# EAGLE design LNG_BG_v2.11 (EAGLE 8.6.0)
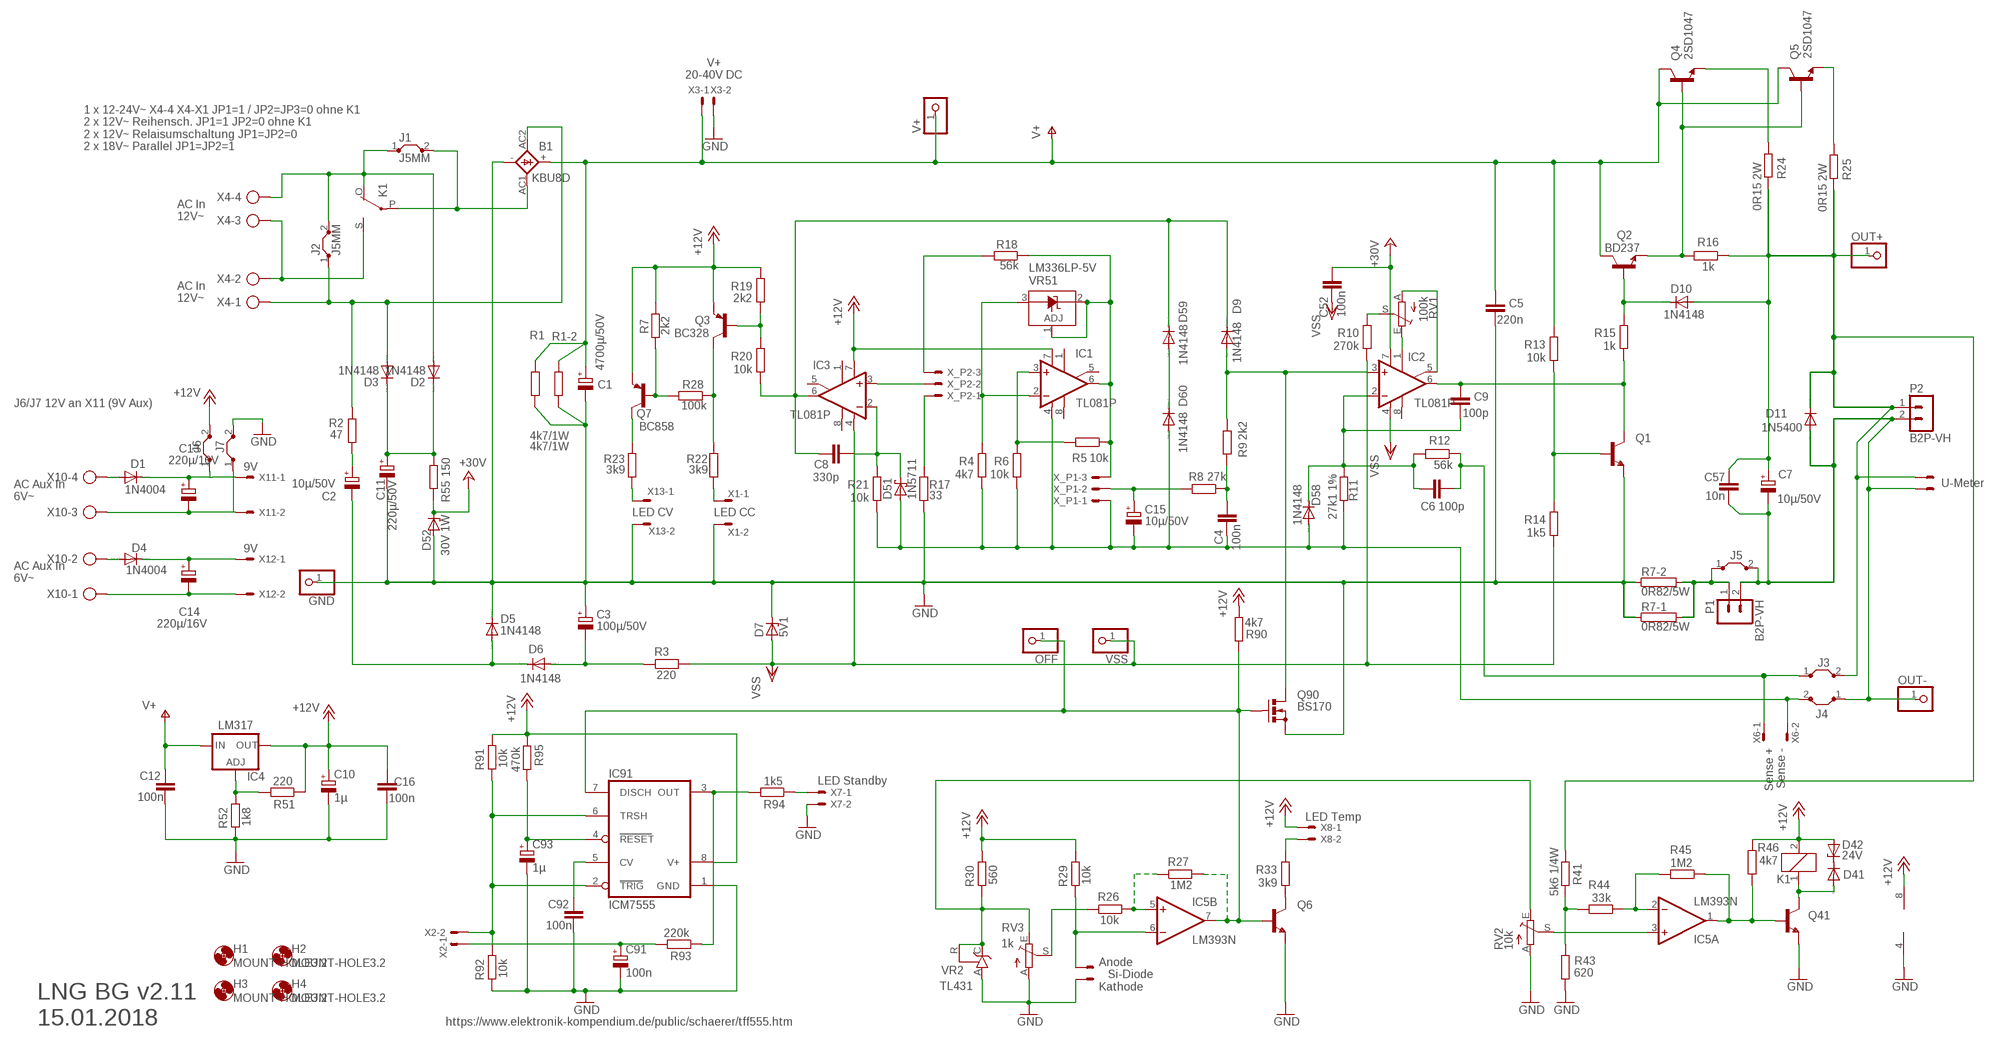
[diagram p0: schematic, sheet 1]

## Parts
B1  KBU8D  GBU4  [GBU4S]
C1  4700µ/50V  CPOL-EUE10-25  [EB25D]
C2  10µ/50V  CPOL-EUE2.5-6  [E2,5-6]
C3  100µ/50V  CPOL-EUE2.5-6  [E2,5-6]
C4  100n  C-EU050-024X044  [C050-024X044]
C5  220n  C-EUC1206  [C1206]
C6  100p  C-EU050-024X044  [C050-024X044]
C7  10µ/50V  CPOL-EUE2.5-6  [E2,5-6]
C8  330p  C-EU050-024X044  [C050-024X044]
C9  100p  C-EU050-024X044  [C050-024X044]
C10  1µ  CPOL-EUE1.8-4  [E1,8-4]
C11  220µ/50V  CPOL-EUE5-10.5  [E5-10,5]
C12  100n  C-EUC0805K  [C0805K]
C13  220µ/16V  CPOL-EUE3.5-8  [E3,5-8]
C14  220µ/16V  CPOL-EUE3.5-8  [E3,5-8]
C15  10µ/50V  CPOL-EUE2.5-6  [E2,5-6]
C16  100n  C-EUC0805  [C0805]
C52  100n  C-EUC0805  [C0805]
C57  10n  C-EUC1206  [C1206]
C91  100n  CPOL-EUE1.8-4  [E1,8-4]
C92  100n  C-EUC0805  [C0805]
C93  1µ  CPOL-EUE1.8-4  [E1,8-4]
D1  1N4004  [DO41-10]
D2  1N4148  1N4004  [DO41-10]
D3  1N4148  1N4004  [DO41-10]
D4  1N4004  [DO41-10]
D5  1N4148  1N4148DO35-10  [DO35-10]
D6  1N4148  1N4148DO35-10  [DO35-10]
D7  5V1  BZV10  [DO34Z7]
D9  1N4148  1N4148DO35-10  [DO35-10]
D10  1N4148  1N4148DO35-10  [DO35-10]
D11  1N5400  [DO201-15]
D41  ES2D  [SMB]
D42  24V  ZENER-DIODESOD80C  [SOD80C]
D51  1N5711  SCHOTTKY-DIODEDO35-7  [DO35-7]
D52  30V 1W  ZPY  [DO41Z10]
D58  1N4148  1N4148DO35-10  [DO35-10]
D59  1N4148  1N4148DO35-10  [DO35-10]
D60  1N4148  1N4148DO35-10  [DO35-10]
GND  PINHD-1X1  [1X01]
H1  MOUNT-HOLE3.2  [3,2]
H2  MOUNT-HOLE3.2  [3,2]
H3  MOUNT-HOLE3.2  [3,2]
H4  MOUNT-HOLE3.2  [3,2]
IC1  TL081P  [DIL08]
IC2  TL081P  [DIL08]
IC3  TL081P  [DIL08]
IC4  LM317  LM317TS  [317TS]
IC5  LM393N  [DIL08]
IC91  ICM7555  [DIL08]
J1  J5MM  [05]
J2  J5MM  [05]
J3  J5MM  [05]
J4  J5MM  [05]
J5  J5MM  [05]
J6  J5MM  [05]
J7  J5MM  [05]
K1  G6RW  [G6RW]
OFF  PINHD-1X1  [1X01]
OUT+  PINHD-1X1  [1X01]
OUT-  PINHD-1X1  [1X01]
P1  B2P-VH  [B2P-VH]
P2  B2P-VH  [B2P-VH]
Q1  BC337-NPN-TO92-CBE  [TO92-CBE]
Q2  BD237  -NPN-TO126V  [TO126V]
Q3  BC328  [TO92-EBC]
Q4  2SD1047  2SC3855  [SC-65]
Q5  2SD1047  2SC3855  [SC-65]
Q6  BC337-NPN-TO92-CBE  [TO92-CBE]
Q7  BC858  BC858ALT1SMD  [SOT23-BEC]
Q41  BC337-NPN-TO92-CBE  [TO92-CBE]
Q90  BS170  [SOT54E]
R1  4k7/1W  R-EU_R2512  [R2512]
R1-2  4k7/1W  R-EU_R2512  [R2512]
R2  47  R-EU_0411/15  [0411/15]
R3  220  R-EU_0207/10  [0207/10]
R4  4k7  R-EU_0207/10  [0207/10]
R5  10k  R-EU_0207/10  [0207/10]
R6  10k  R-EU_0207/10  [0207/10]
R7  2k2  R-EU_R1206  [R1206]
R7-1  0R82/5W  RKH208-8  [KH208-8]
R7-2  0R82/5W  RKH208-8  [KH208-8]
R8  27k  R-EU_0207/10  [0207/10]
R9  2k2  R-EU_0207/10  [0207/10]
R10  270k  R-EU_0207/10  [0207/10]
R11  27k1 1%  R-EU_0207/10  [0207/10]
R12  56k  R-EU_0207/10  [0207/10]
R13  10k  R-EU_0207/10  [0207/10]
R14  1k5  R-EU_0207/10  [0207/10]
R15  1k  R-EU_0207/10  [0207/10]
R16  1k  R-EU_0207/10  [0207/10]
R17  33  R-EU_0207/10  [0207/10]
R18  56k  R-EU_0207/10  [0207/10]
R19  2k2  R-EU_0207/10  [0207/10]
R20  10k  R-EU_0207/10  [0207/10]
R21  10k  R-EU_0207/10  [0207/10]
R22  3k9  R-EU_0207/10  [0207/10]
R23  3k9  R-EU_0207/10  [0207/10]
R24  0R15 2W  R-EU_0617/5V  [0617V]
R25  0R15 2W  R-EU_0617/5V  [0617V]
R26  10k  R-EU_0207/10  [0207/10]
R27  1M2  R-EU_0207/10  [0207/10]
R28  100k  R-EU_R1206  [R1206]
R29  10k  R-EU_0207/10  [0207/10]
R30  560  R-EU_0207/10  [0207/10]
R33  3k9  R-EU_0207/10  [0207/10]
R41  5k6 1/4W  R-EU_0207/10  [0207/10]
R43  620  R-EU_0207/10  [0207/10]
R44  33k  R-EU_0207/10  [0207/10]
R45  1M2  R-EU_0207/10  [0207/10]
R46  4k7  R-EU_0207/10  [0207/10]
R51  220  R-EU_0207/10  [0207/10]
R52  1k8  R-EU_0207/10  [0207/10]
R55  150  R-EU_0207/10  [0207/10]
R90  4k7  R-EU_0207/10  [0207/10]
R91  10k  R-EU_0207/10  [0207/10]
R92  10k  R-EU_0207/10  [0207/10]
R93  220k  R-EU_0207/10  [0207/10]
R94  1k5  R-EU_0207/10  [0207/10]
R95  470k  R-EU_0207/10  [0207/10]
RV1  100k  TRIM_EU-B64Y  [B64Y]
RV2  10k  TRIM_EU-B64Y  [B64Y]
RV3  1k  TRIM_EU-B64Y  [B64Y]
U_METER  U-Meter  22-23-2021  [22-23-2021]
V+  PINHD-1X1  [1X01]
VR2  TL431  TL431CLP  [TO92-CLP]
VR51  LM336LP-5V  LM336LP  [TO92]
VSS  PINHD-1X1  [1X01]
X1  LED CC  22-23-2021  [22-23-2021]
X2  PSK-2  22-23-2021  [22-23-2021]
X3  PSK-2  22-23-2021  [22-23-2021]
X4  AK500/4  [AK500/4]
X5  PSK-2  22-23-2021  [22-23-2021]
X6  22-23-2021  [22-23-2021]
X7  LED Standby  22-23-2021  [22-23-2021]
X8  LED Temp  22-23-2021  [22-23-2021]
X10  AK500/4  [AK500/4]
X11  9V  22-23-2021  [22-23-2021]
X12  9V  22-23-2021  [22-23-2021]
X13  LED CV  22-23-2021  [22-23-2021]
X_P1  22-23-2031  [22-23-2031]
X_P2  22-23-2031  [22-23-2031]

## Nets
+12V: C10.+ C16.1 D42.A IC1.7(V+) IC3.7(V+) IC4.2(OUT) IC5.8(P:V+) IC91.8(V+) J6.2 K1.2 Q3.E Q7.E R7.1 R19.2 R29.2 R30.2 R46.2 R51.1 R90.1 R91.2 R95.1 X8.1
+24V: C52.1 D52.C IC2.7(V+) R55.1 ; supply symbol labelled +30V
AC2-1: K1.S(2:S) X4.2 X4.3
AC2-2: B1.AC2(AC1) D3.A J2.1 R2.1 X4.1
GND: B1.- C1.- C3.+ C5.2 C10.- C11.- C12.2 C16.2 C91.- C92.2 C93.- D5.C D7.C D52.A GND.1 IC5.4(P:V-) IC91.1(GND) J7.2 Q1.E Q6.E Q41.E Q90.S R1-2.1 R1.1 R7-1.1 R7-2.1 R17.1 R43.1 R52.1 R92.1 RV2.A RV3.A VR2.A X1.2 X3.2 X5.2 X7.2 X13.2
N$1: IC91.3(OUT) R93.1 R94.2
N$2: R94.1 X7.1
N$3: C2.+ R2.2
N$4: B1.AC1(AC2) J1.2 K1.P(2:P)
N$5: C2.- D5.A D6.C
N$6: Q3.B R19.1 R20.2
N$7: C3.- D6.A R3.1
N$8: D59.A D60.C
N$9: C8.2 D9.C D59.C IC3.6(OUT) R20.1
N$10: C8.1 D51.C IC3.2(-IN) R21.2
N$11: R22.1 X1.1
N$12: Q3.C R22.2 R28.1
N$13: C11.+ D2.C D3.C R55.2
N$14: IC3.3(+IN) X_P2.2
N$15: R17.2 X_P2.1
N$16: R18.2 X_P2.3
N$17: IC1.3(+IN) R5.2 R6.2
N$18: R41.1 R43.2 R44.2
N$19: IC1.2(-IN) R4.2 VR51.3(A)
N$20: J5.1 P1.1 R7-1.2 R7-2.2
N$21: C4.1 R8.1 R9.2
N$22: D9.A IC2.3(+IN) Q90.D R9.1
N$23: C93.+ IC91.4(RESET) R95.2
N$24: R10.2 RV1.S
N$25: IC2.1(ON1) RV1.E
N$26: IC2.5(ON2) RV1.A
N$27: C9.1 IC2.6(OUT) Q1.C R15.1
N$28: Q1.B R13.1 R14.2
N$29: D10.C Q2.3(B) R15.2
N$30: IC5.2(A:-IN) R44.1 R45.2
N$31: IC5.5(B:+IN) R26.2 R27.1
N$32: IC91.2(TRIG) IC91.6(TRSH) R91.1 R92.2 X2.2
N$33: IC5.3(A:+IN) RV2.S
N$34: C15.+ R8.2 X_P1.2
N$35: C6.1 C9.2 D58.C IC2.2(-IN) R11.2 R12.2
N$36: C92.1 IC91.5(CV)
N$37: IC5.6(B:-IN) R29.1 X5.1
N$38: R33.2 X8.2
N$39: IC5.1(A:OUT) Q41.B R45.1 R46.1
N$40: R30.1 RV2.E RV3.E VR2.C VR2.R
N$41: D41.A K1.1 Q41.C
N$42: Q4.3(E) R24.2
N$43: C13.+ D1.C J6.1 X11.1
N$44: IC4.1(ADJ) R51.2 R52.2
N$45: R26.1 RV3.S
N$46: D2.A J1.1 J2.2 K1.O(2:O) X4.4
N$47: Q5.3(E) R25.2
N$48: R23.1 X13.1
N$49: Q7.B R7.2 R28.2
N$50: Q2.1(E) Q4.1(B) Q5.1(B) R16.2
N$51: C14.+ D4.C X12.1
N$52: D1.A X10.4
N$53: C91.+ R93.2 X2.1
N$54: Q7.C R23.2
N$55: D4.A X10.2
N$56: Q6.C R33.1
N$57: C13.- J7.1 X10.3 X11.2
N$59: C14.- X10.1 X12.2
N$60: D41.C D42.C
OUT+: C7.+ C57.2 D10.A D11.C J3.2 OUT+.1 P2.1 R16.1 R24.1 R25.1 R41.2 U_METER.1
OUT-: C7.- C57.1 D11.A J4.1 J5.2 OUT-.1 P1.2 P2.2 U_METER.2
SENSE+: C6.2 J3.1 R12.1 X6.1
SENSE-: C4.2 C15.- D51.A D58.A D60.A IC1.4(V-) J4.2 R4.1 R6.1 R11.1 R21.1 X6.2 X_P1.1
SHUTDOWN: IC5.7(B:OUT) IC91.7(DISCH) OFF.1 Q6.B Q90.G R27.2 R90.2
V+: B1.+ C1.+ C5.1 C12.1 IC4.3(IN) Q2.2(C) Q4.2(C) Q5.2(C) R1-2.2 R1.2 R13.2 V+.1 X3.1
VREF: IC1.6(OUT) R5.1 R18.1 VR51.1(ADJ) VR51.2(C) X_P1.3
VSS: C52.2 D7.A IC2.4(V-) IC3.4(V-) R3.2 R10.1 R14.1 VSS.1
Unconnected: IC1.1(ON1) IC1.5(ON2) IC1.8(OPT) IC2.8(OPT) IC3.1(ON1) IC3.5(ON2) IC3.8(OPT)

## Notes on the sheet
- V+
  20-40V DC
- 1 x 12-24V~ X4-4 X4-X1 JP1=1 / JP2=JP3=0 ohne K1
  2 x 12V~ Reihensch. JP1=1 JP2=0 ohne K1
  2 x 12V~ Relaisumschaltung JP1=JP2=0
  2 x 18V~ Parallel JP1=JP2=1
- AC In
  12V~
- AC In
  12V~
- J6/J7 12V an X11 (9V Aux)
- AC Aux In
  6V~
- AC Aux In
  6V~
- Sense +
  Sense -
- Anode
     Si-Diode
  Kathode
- LNG BG v2.11
  15.01.2018
- https://www.elektronik-kompendium.de/public/schaerer/tff555.htm

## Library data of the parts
B1 = rectifier:GBU4: GENERAL INSTRUMENT RECTIFIER
C1-C3 C7 C10 C11 C13-C15 C91 C93 = rcl:CPOL-EU: POLARIZED CAPACITOR, European symbol; SPICEPREFIX: C
C4-C6 C8 C9 C12 C16 C52 C57 C92 = rcl:C-EU: CAPACITOR, European symbol; SPICEPREFIX: C
D1-D4 = diode:1N4004: DIODE
D5 D6 D9 D10 D58-D60 = diode:1N4148: DIODE
D7 = diode:BZV10: Z DIODE
D11 = diode:1N5400: DIODE
D41 = diode:ES2D: DIODE
D42 = diode:ZENER-DIODE: Z-Diode
D51 = diode:SCHOTTKY-DIODE: Schottky Diode
D52 = diode:ZPY: Z DIODE
GND OFF OUT+ OUT- V+ VSS = pinhead:PINHD-1X1: PIN HEADER
H1-H4 = holes:MOUNT-HOLE: MOUNTING HOLE with drill center marker
IC1-IC3 = linear:TL081: OP AMP
IC4 = v-reg:LM317TS: VOLTAGE REGULATOR
IC5 = linear:LM393: COMPARATOR
IC91 = maxim:ICM7555: TIMER; MF: MAXIM; MPN: ICM7555IPA+; OC_FARNELL: 9663762; OC_NEWARK: 68K4387
J1-J7 = jumper:J: Bridge
K1 = relay:G6RW: RELAY 1 x switch, Omron; OC_FARNELL: unknown; OC_NEWARK: unknown
P1 P2 = con-jst-vh:B2P-VH: HEADER
Q1 Q2 Q6 Q41 = transistor:*-NPN-: NPN Transistror BF959 corrected 2008.03.06
Q3 = transistor-pnp:BC328*: PNP Transistror
Q4 Q5 = transistor-JP:2SC3855: NPN Power Transistor 140V, 10A, 100W
Q7 = transistor-pnp:BC858*: PNP Transistror
Q90 = transistor-small-signal:BS170: N-CHANNEL MOS FET
R1 R1-2 R2-R30 R33 R41 R43-R46 R51 R52 R55 R90-R95 = rcl:R-EU_: RESISTOR, European symbol; SPICEPREFIX: R
R7-1 R7-2 = resistor-power:R: Power Resitor; OC_FARNELL: unknown; OC_NEWARK: unknown
RV1-RV3 = pot:TRIM_EU-: POTENTIOMETER
U_METER X1-X3 X5-X8 X11-X13 = con-molex:22-23-2021: .100" (2.54mm) Center Header - 2 Pin; MF: MOLEX; MPN: 22-23-2021; OC_FARNELL: 1462926; OC_NEWARK: 25C3832
VR2 = v-reg:TL431CLP: VOLTAGE REGULATOR
VR51 = linear:LM336: 2.5-V INTEGRATED REFERENCE CIRCUITS LM236 Source: http://focus.ti.com/lit/ds/symlink/lm336-2.5.pdf
X4 X10 = con-ptr500:AK500/4: CONNECTOR; OC_FARNELL: unknown; OC_NEWARK: unknown
X_P1 X_P2 = con-molex:22-23-2031: .100" (2.54mm) Center Header - 3 Pin; MF: MOLEX; MPN: 22-23-2031; OC_FARNELL: 1462950; OC_NEWARK: 30C0862

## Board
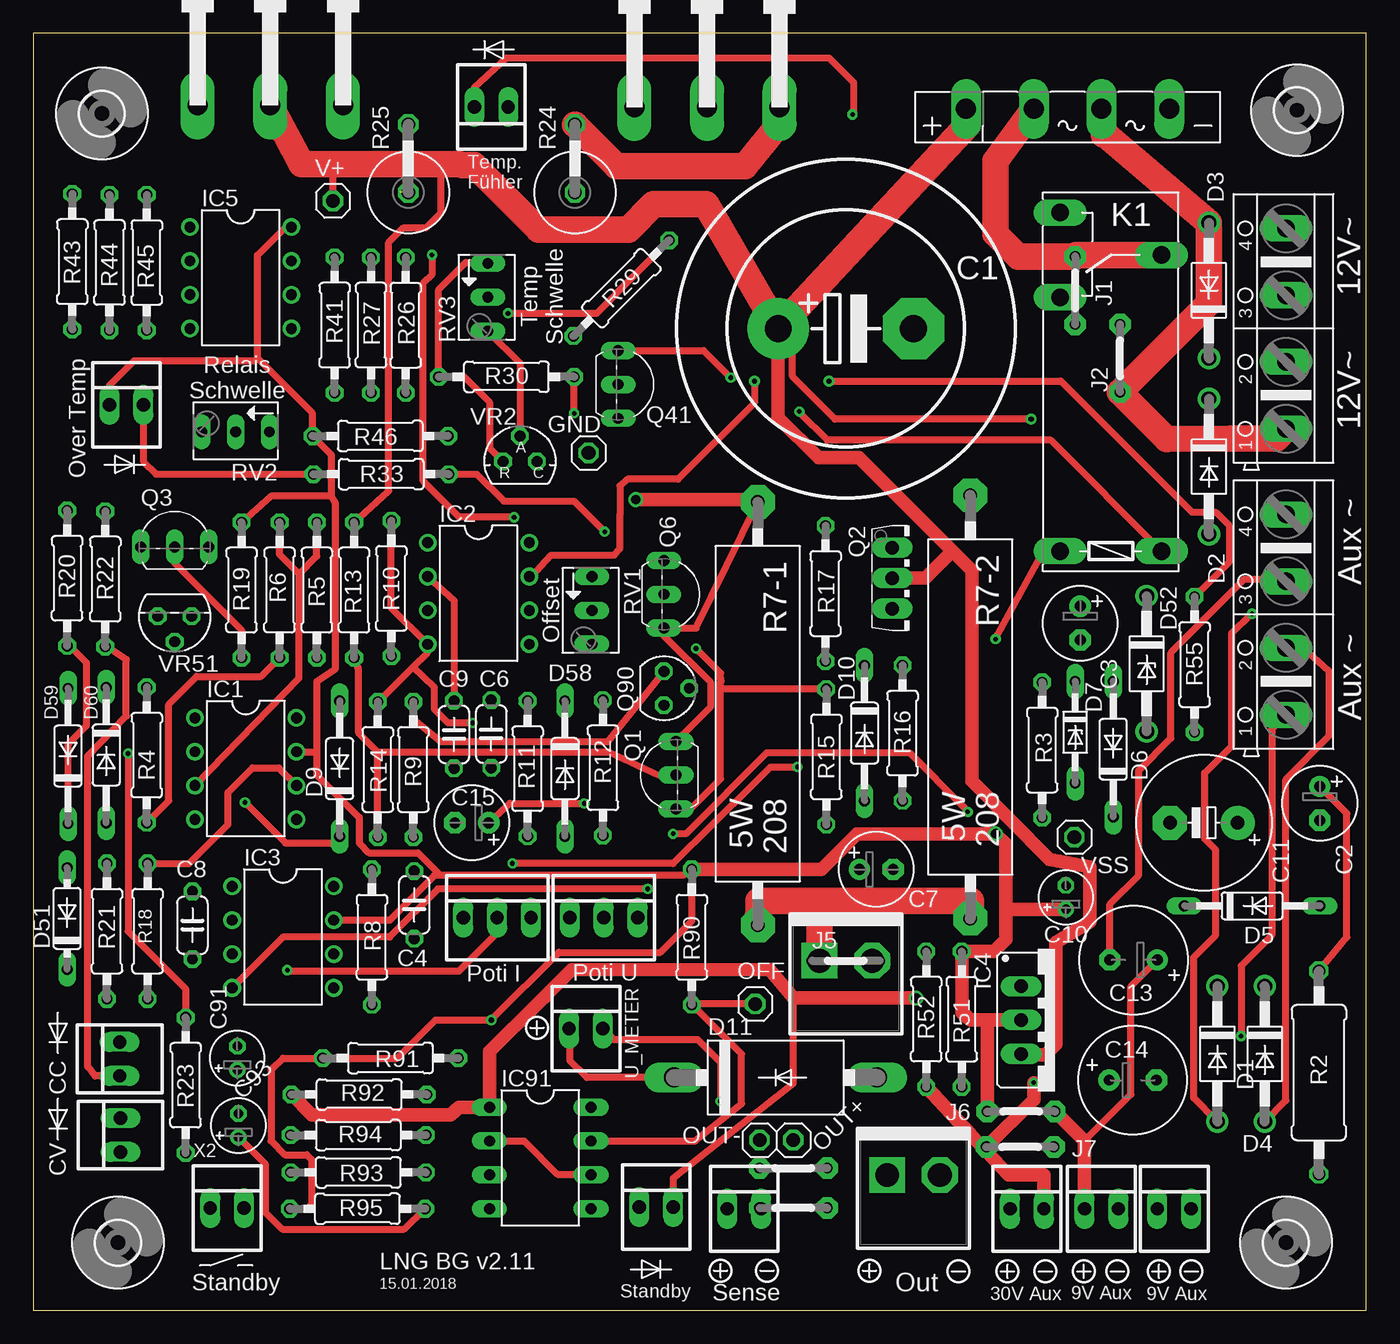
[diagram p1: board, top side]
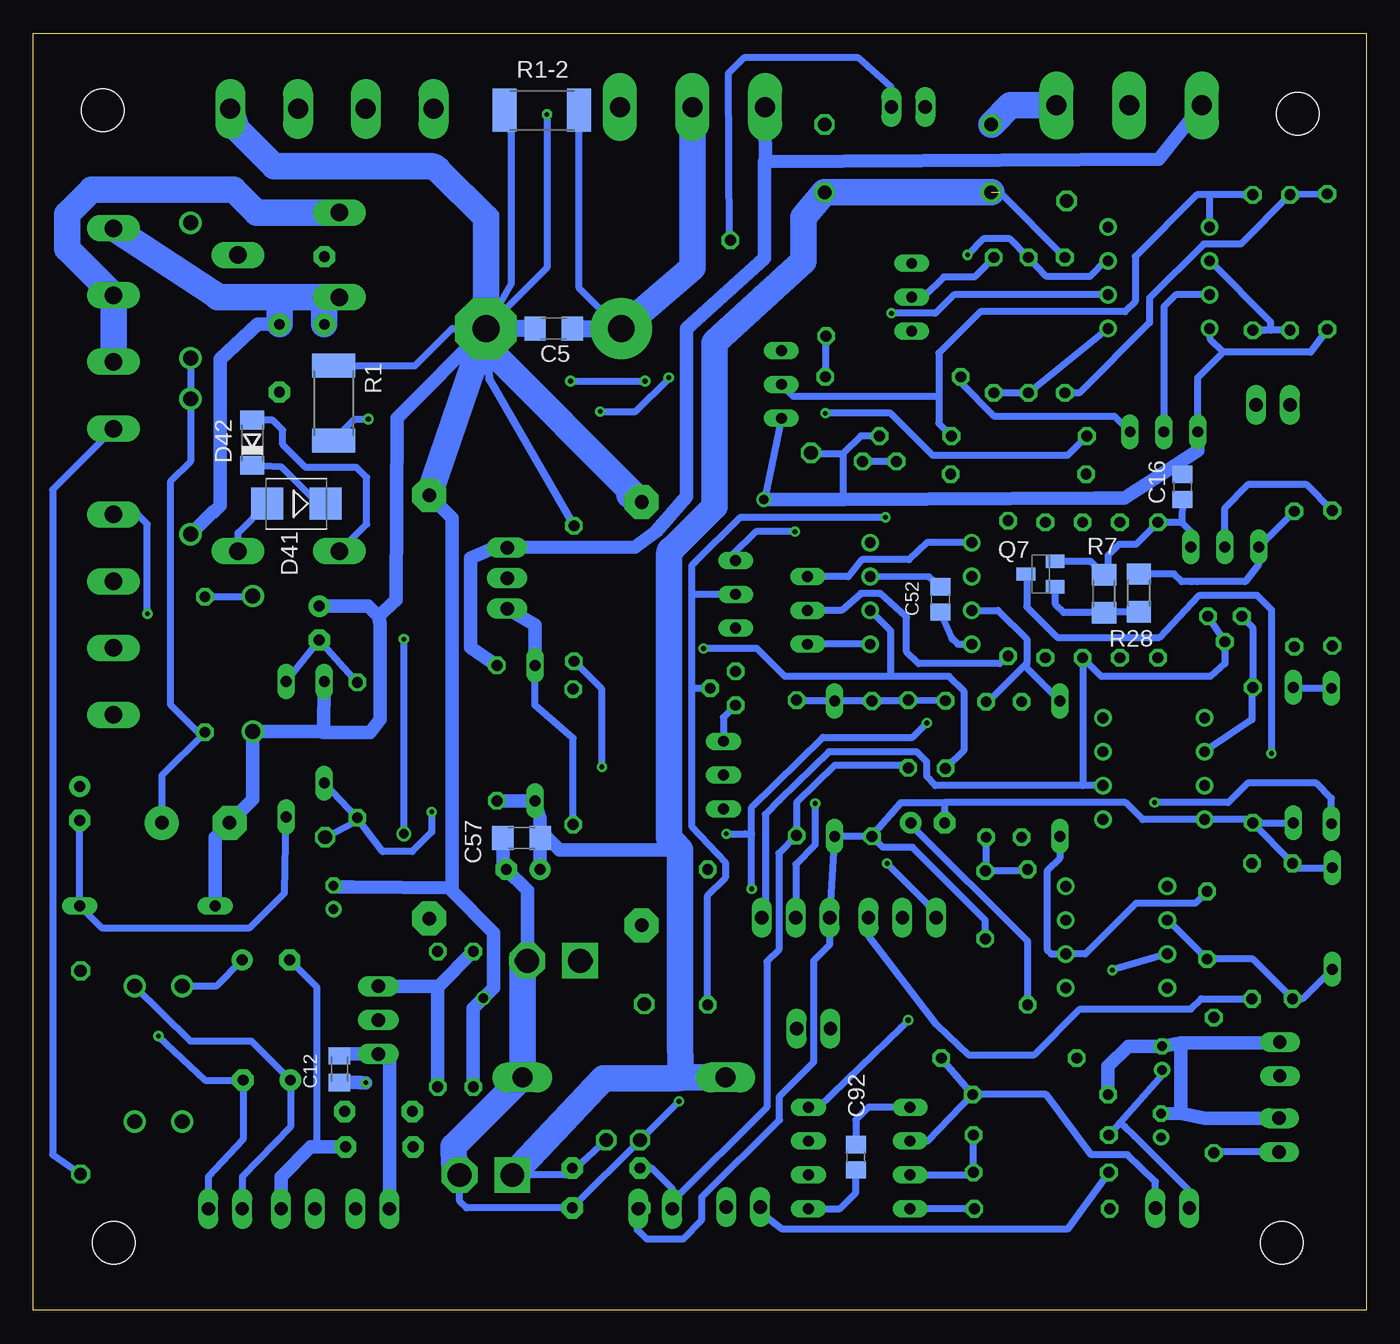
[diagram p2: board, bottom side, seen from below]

Size 100 x 95.81 mm. Coordinates in mm from the lower left corner, seen from the top.
Outline: 0,0 100,0 100,95.81 0,95.81 0,0
Copper layers (1*16): Top 0.035mm / dielectric 1.5mm / Bottom 0.035mm
Design rules "default *": minimum track width 6mil, minimum drill 0.35mm, track to track 10mil, track to pad 10mil, pad to pad 10mil, via to via 15mil, smd to smd 6mil, copper to edge 40mil, drill to drill 6mil, minimum pad ring 10mil, minimum via ring 8mil, stop-mask expansion 4mil, vias tented up to drill 0mil, thermal gap 10mil

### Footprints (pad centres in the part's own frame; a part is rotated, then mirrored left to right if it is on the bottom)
GBU4S = drill 1.499 long: + 7.62,0; - -7.62,0; AC1 2.54,0; AC2 -2.54,0
EB25D = drill 2.007 pad 4.597: + -5.08,0 | drill 2.007 pad 4.597 octagon: - 5.08,0
E2,5-6 = drill 0.813 pad 1.6: + -1.27,0 | drill 0.813 pad 1.6 octagon: - 1.27,0
C050-024X044 = drill 0.813 octagon: 1 -2.54,0; 2 2.54,0
C1206 = smd 1.6 x 1.8: 1 -1.4,0; 2 1.4,0
E1,8-4 = drill 0.711 pad 1.168: + -0.889,0 | drill 0.711 pad 1.168 octagon: - 0.889,0
E5-10,5 = drill 1.016 pad 2.54: + -2.54,0 | drill 1.016 pad 2.54 octagon: - 2.54,0
C0805K = smd 1.3 x 1.6: 1 -1,0; 2 1,0
E3,5-8 = drill 0.813 pad 1.6: + -1.778,0 | drill 0.813 pad 1.6 octagon: - 1.778,0
C0805 = smd 1.3 x 1.5: 1 -0.95,0; 2 0.95,0
DO41-10 = drill 1.118: A 5.08,0; C -5.08,0
DO35-10 = drill 0.813 long: A 5.08,0; C -5.08,0
DO34Z7 = drill 0.813 long: A 3.81,0; C -3.81,0
DO201-15 = drill 1.499 long: A 7.62,0; C -7.62,0
SMB = smd 2.4 x 2.4: A 2.2,0; C -2.2,0
SOD80C = smd 1.4 x 1.8: A 1.7,0; C -1.7,0
DO35-7 = drill 0.813 long: A 3.81,0; C -3.81,0
DO41Z10 = drill 1.118: A 5.08,0; C -5.08,0
1X01 = drill 1.016 octagon: 1 0,0
3,2 = hole 3.2: 0,0
DIL08 = drill 0.813 pad 1.27: 1 -3.81,-3.81; 2 -1.27,-3.81; 3 1.27,-3.81; 4 3.81,-3.81; 5 3.81,3.81; 6 1.27,3.81; 7 -1.27,3.81; 8 -3.81,3.81
317TS = drill 1.016 long: 1 -2.54,-2.54; 2 0,-2.54; 3 2.54,-2.54
DIL08' = drill 0.813 long: 1 -3.81,-3.81; 2 -1.27,-3.81; 3 1.27,-3.81; 4 3.81,-3.81; 5 3.81,3.81; 6 1.27,3.81; 7 -1.27,3.81; 8 -3.81,3.81
05 = drill 0.813 pad 1.6 octagon: 1 -2.54,0; 2 2.54,0
G6RW = drill 1.321 long: 1 -12.7,-3.81; 2 -12.7,3.81; O 6.35,3.81; P 9.525,-3.81; S 12.7,3.81
B2P-VH = drill 1.778 square: 1 -1.98,0 | drill 1.778 octagon: 2 1.98,0
TO92-CBE = drill 0.813 long: B 0,0; C -2.54,0; E 2.54,0
TO126V = drill 1.016 long: 1 -2.286,-1.27; 2 0,-1.27; 3 2.286,-1.27
TO92-EBC = drill 0.813 long: B 0,-1.27; C -2.54,-1.27; E 2.54,-1.27
SC-65 = drill 1.5 pad 2.54 long: 1 -5.45,-18.81; 2 0,-18.81; 3 5.45,-18.81
SOT23-BEC = smd 1 x 1.4: B -0.95,-1.1; C 0,1.1; E 0.95,-1.1
SOT54E = drill 0.813 octagon: D -1.27,0; G 0,1.905; S 1.27,0
R2512 = smd 1.8 x 3.2: 1 -2.8,0; 2 2.8,0
0411/15 = drill 0.914 octagon: 1 -7.62,0; 2 7.62,0
0207/10 = drill 0.813 octagon: 1 -5.08,0; 2 5.08,0
R1206 = smd 1.6 x 1.803: 1 -1.422,0; 2 1.422,0
KH208-8 = drill 1.016 pad 2.54 octagon: 1 -15.875,0; 2 15.875,0
0617V = drill 1.016 octagon: 1 -2.54,0; 2 2.54,0
B64Y = drill 0.813 long: A 2.54,0; E -2.54,0; S 0,0
22-23-2021 = drill 1 long: 1 -1.27,0; 2 1.27,0
TO92-CLP = drill 0.813 octagon: A 0,1.905; C 1.27,0; R -1.27,0
TO92 = drill 0.813 octagon: 1 -1.27,0; 2 0,1.905; 3 1.27,0
AK500/4 = drill 1.321 long: 1 -7.518,0; 2 -2.489,0; 3 2.489,0; 4 7.518,0
22-23-2031 = drill 1 long: 1 -2.54,0; 2 0,0; 3 2.54,0

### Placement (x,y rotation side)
B1  77.61,90.15 180 top
C1  60.96,73.66 0 top
C2  96.52,38.04 270 top
C3  78.55,51.56 270 top
C4  28.57,30.42 270 top
C5  60.96,73.66 180 bottom
C6  34.35,43.24 270 top
C7  63.25,33.08 0 top
C8  11.94,28.89 90 top
C9  31.56,43.2 90 top
C10  77.47,30.99 90 top
C11  87.82,36.58 180 top
C12  77.03,18.1 270 bottom
C13  82.55,26.29 180 top
C14  82.49,17.27 0 top
C15  32.89,36.58 180 top
C16  13.78,61.78 90 bottom
C52  31.94,53.34 270 bottom
C57  63.37,35.43 0 bottom
C91  15.3,18.92 90 top
C92  38.29,11.49 90 bottom
C93  15.39,13.87 90 top
D1  88.84,19.24 270 top
D2  88.2,63.31 270 top
D3  88.2,76.52 90 top
D4  92.39,19.24 270 top
D5  91.44,30.35 0 top
D6  81.03,42.1 90 top
D7  78.17,43.37 270 top
D9  22.99,40.64 90 top
D10  62.36,43.31 270 top
D11  55.69,17.46 0 top
D41  80.26,60.52 180 bottom
D42  83.57,65.09 90 bottom
D51  2.54,29.4 90 top
D52  83.53,48.51 270 top
D58  39.88,40.64 270 top
D59  2.6,41.59 90 top
D60  5.46,41.66 270 top
GND  41.66,64.33 0 top
H1  5.14,89.79 0 top
H2  6.35,5.08 0 top
H3  93.98,5.08 0 top
H4  94.81,90.04 0 top
IC1  15.94,40.64 270 top
IC2  33.4,53.78 270 top
IC3  18.73,28 270 top
IC4  76.64,21.78 270 top
IC5  15.56,77.47 270 top
IC91  ICM7555  [DIL08']  38.04,11.43 270 top
J1  78.17,76.52 90 top
J2  81.53,71.44 90 top
J3  57.02,10.67 0 top
J4  57.02,7.68 180 top
J5  60.96,26.23 0 top
J6  74.1,14.92 180 top
J7  74.04,12.26 180 top
K1  80.84,69.66 90 top
OFF  54.17,22.99 0 top
OUT+  57.02,12.76 0 top
OUT-  54.48,12.76 0 top
P1  60.96,26.23 0 top
P2  66.04,10.16 0 top
Q1  48.22,40.16 90 top
Q2  65.72,54.93 270 top
Q3  10.6,58.55 0 top
Q4  50.55,109.09 0 top
Q5  17.78,109.22 0 top
Q6  47.31,53.72 270 top
Q7  24.43,55.24 90 bottom
Q41  43.88,69.47 270 top
Q90  47.31,46.67 270 top
R1  77.47,68.07 270 bottom
R1-2  61.85,90.04 0 bottom
R2  96.46,17.84 90 top
R3  75.69,42.04 270 top
R4  8.51,41.66 90 top
R5  21.27,54.04 90 top
R6  18.48,54.04 90 top
R7  19.66,53.76 270 bottom
R7-1  54.36,44.77 270 top
R7-2  70.29,45.28 270 top
R8  25.4,28 270 top
R9  28.51,40.58 270 top
R10  26.86,54.17 270 top
R11  37.08,40.64 90 top
R12  42.74,40.7 90 top
R13  24.07,54.04 90 top
R14  25.84,40.58 270 top
R15  59.5,41.53 270 top
R16  65.21,43.31 90 top
R17  59.44,53.78 270 top
R18  8.57,28.45 270 top
R19  15.62,54.04 90 top
R20  2.54,54.93 90 top
R21  5.52,28.45 270 top
R22  5.4,54.86 90 top
R23  11.43,16.89 90 top
R24  40.64,86.42 90 top
R25  28.13,86.42 90 top
R26  27.94,73.91 270 top
R27  25.34,73.91 90 top
R28  17.06,53.82 270 bottom
R29  44.11,76.69 225 top
R30  35.5,70.04 0 top
R33  26.1,62.74 180 top
R41  22.61,73.91 90 top
R43  2.92,78.68 90 top
R44  5.71,78.61 90 top
R45  8.51,78.61 270 top
R46  26.04,65.6 180 top
R51  69.66,21.84 270 top
R52  66.99,21.84 90 top
R55  87.12,48.45 270 top
R90  49.4,28 270 top
R91  26.8,18.92 180 top
R92  24.45,16.19 0 top
R93  24.38,13.14 180 top
R94  24.38,10.35 0 top
R95  24.32,7.62 0 top
RV1  41.91,52.51 270 top
RV2  15.18,65.91 180 top
RV3  34.1,76.01 270 top
U_METER  41.47,21.15 0 top
V+  22.48,83.25 0 top
VR2  36.51,63.69 0 top
VR51  10.6,52.07 180 top
VSS  78.11,35.5 0 top
X1  6.48,18.86 90 top
X2  14.54,7.68 0 top
X3  74.55,7.62 0 top
X4  93.98,73.66 90 top
X5  34.35,90.3 180 top
X6  53.34,7.62 0 top
X7  46.74,7.75 0 top
X8  6.99,67.95 0 top
X10  93.98,52.2 90 top
X11  80.14,7.62 0 top
X12  85.6,7.62 0 top
X13  6.54,13.14 90 top
X_P1  42.8,29.46 0 top
X_P2  34.8,29.46 0 top

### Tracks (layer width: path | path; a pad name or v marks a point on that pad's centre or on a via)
+12V  (via drill 0.35, 0.4, 0.7)
  Top 0.508: 77.09,56.83 K1.2 75.56,56.52 v72.2,50.36 | 16.83,71.44 20.95,67.31 R46.2 22.35,64.2 22.35,61.09 | 16.83,71.44 16.83,79.18 18.92,81.28 IC5.8 | X8.1 5.71,69.41 7.56,71.25 16.64,71.25 16.83,71.44 | 22.35,61.09 17.84,61.09 R19.2 | 30.54,32.64 48.77,32.64 R90.1 49.4,29.21 47.05,26.86 39.43,26.86 v34.35,21.78 30.16,21.78 27.3,18.92 R91.2 18.73,18.92 17.84,18.03 17.84,12.7 18.86,11.68 20.51,11.68 20.89,11.3 20.89,7.94 20.57,7.62 R95.1 | 30.54,32.64 30.1,32.64 26.73,29.27 IC3.7 | 22.35,61.09 22.67,60.58 22.67,48.13 21.27,47.18 21.27,41.97 | v72.2,35.75 71.12,35.75 | IC1.7 21.21,41.91 21.27,41.97 | 21.27,41.97 21.27,40.16 24.45,36.98 24.45,35.05 25.17,34.33 28.86,34.33 29.74,33.44 30.54,32.64 | v40.58,67.31 R30.2
  Top 1.016: 71.44,35.76 v72.19,35.75 71.12,35.75 61.79,35.75 59.12,33.08 R90.1 | IC4.2 71.63,21.78 | 71.63,21.78 70.29,21.78 69.66,22.35 R51.1 72.07,26.92 72.96,27.81 72.96,30.1 | C10.+ 72.96,30.1 | v72.2,35.75 72.96,34.99 72.96,30.1 | J6.2 71.56,21.72 71.63,21.78
  Bottom 0.508: 76.71,57.4 K1.2 74.99,58.99 74.99,62.48 75.75,63.25 79.57,63.25 81.28,64.96 81.28,66.04 82.03,66.79 D42.A | v34.35,21.78 34.92,21.21 41.15,15.18 IC91.8 42.23,15.24 | R29.2 40.58,73.03 R30.2 | Q3.E 13.14,58.42 13.84,59.12 | 13.84,59.12 R19.2 17.27,57.47 18.54,57.47 19.37,56.64 19.37,55.63 19.66,55.33 R7.1 20.67,56.19 Q7.E | v72.2,35.75 v72.2,50.36 | C16.1 13.84,59.12 | R46.2 22.42,64.14 32.51,64.14 35.69,67.31 v40.58,67.31
+24V  (via drill 0.4)
  Top 0.508: v59.69,69.72 77.09,69.72 86.93,59.88 88.71,59.88 89.72,58.86 89.72,56.13 R55.1 | v54.1,69.72 54.1,68.07 48.39,62.36 44.58,62.36 44.01,61.85 44.01,59.69 44.01,58.49 44.01,58.42 44.01,57.15 43.59,56.67 38.86,56.67 37.38,55.05 IC2.7
  Bottom 0.508: v59.69,69.72 v54.1,69.72 | C52.1 32.79,55.03 IC2.7 | D52.C 83.59,53.53 R55.1
AC2-1
  Bottom 2: X4.2 X4.3 97.47,79.64 97.47,82.23 95.63,84.07 84.96,84.07 83.25,82.36 K1.S
AC2-2
  Top 0.508: 95.38,66.04 93.88,66.04 93.24,65.41
  Top 2: X4.1 93.24,65.41 89.85,65.41 85.05,65.38 J2.1 88.2,75.56 D3.A 80.33,88.33 80.34,88.19 B1.AC2
  Bottom 0.508: X4.1 98.55,61.57 98.55,11.68 R2.1
GND  (via drill 0.35, 0.7)
  Top 0.508: 53.85,60.83 R7-1.1 49.72,51.18 Q6.E | X5.2 33.08,91.75 35.5,93.97 59.7,93.97 61.53,92.14 61.53,89.85 61.47,89.79 v61.47,89.73 | Q6.E 47.37,50.86 | RV3.A 36.51,71.06 VR2.A | 57.02,23.43 57.02,17.02 48.01,9.91 X7.2 | Q6.E 47.31,50.61 50.79,47.13 50.79,47.11 50.79,45.27 Q1.E
  Top 1.016: v45.2,60.83 53.85,60.83 | X3.2 75.82,10.16 73.15,10.16 70.94,12.53 | R92.1 20.89,14.67 31.3,14.67 31.94,15.24 IC91.1 34.23,19.43 37.91,23.06 | 37.91,23.06 38.54,23.69 | v66.23,23.43 57.02,23.43 55.24,25.59 40.38,25.53 37.91,23.06 | R52.1 70.3,13.22 70.94,12.53 | 70.94,12.53 71.22,12.53 J7.2 75.06,15.81 v75.06,17.08
  Bottom 0.508: 65.31,82.27 arc45 66.02,81.98 66.04,81.98 | R1.1 71.37,70.87 68.58,73.66 C1.- | 64.58,75.12 C1.- | v61.47,89.73 61.47,78.23 C1.- | R43.1 4.19,71.88 10.73,71.88 | Q41.E 45.15,60.83 | 10.73,71.88 11.68,72.84 11.68,73.6 IC5.4 | RV2.A 12.64,69.98 10.73,71.88 | Q90.S 48.22,44.49 Q1.E | VR2.A 37.91,65.59 39.24,64.26 | 39.24,64.26 39.24,60.9 39.18,60.83 | GND.1 41.59,64.26 39.24,64.26 | IC91.1 37.34,15.24 38.29,14.29 C92.2 | C1.- 64.14,77.03 64.14,88.33 R1-2.1 | C16.2 14.35,63.37 | C93.- 15.23,14.76
  Bottom 0.61: R17.1 65.79,69.85 C1.-
  Bottom 1.016: 54.36,60.99 R7-1.1 | C1.- 72.71,66.93 72.77,53.35 | 72.77,53.35 72.77,53.28 | RV2.A 12.64,64.52 14.35,63.37 18.16,60.96 20.32,60.96 39.18,60.83 45.15,60.83 v45.2,60.83 | R92.1 19.37,18.29 17.84,19.81 C91.- 13.91,20.07 | 13.91,20.07 13.91,14.79 | 13.91,14.79 15.23,14.76 C93.- | X1.2 6.86,20.13 7.87,20.07 13.91,20.07 | R52.1 66.99,22.67 v66.23,23.43 65.47,24.19 65.47,28.32 68.64,31.56 68.58,31.56 68.58,31.69 | R7-2.1 68.58,59.44 68.58,31.69 | C10.- 77.22,31.75 76.07,31.75 68.58,31.69 | 72.77,53.35 74.08,52.04 | 74.08,52.04 73.98,51.5 73.98,49.22 73.98,48.7 73.98,44.32 74.74,43.37 78.23,43.37 | 85.28,36.89 C11.- | C11.- 86.36,35.5 D5.C | X13.2 12.08,14.41 13.91,14.79 | C3.+ 74.87,52.83 74.08,52.04 | 78.23,43.37 D7.C | C11.- 83.53,38.33 D52.A 78.55,43.43 78.23,43.37 | 71.69,12.45 J7.2 | C12.2 75.45,17.1 75.44,17.08 v75.06,17.08
  Bottom 1.27: C5.2 C1.-
  Bottom 2: C1.- 66.04,81.98 69.62,85.56 arc-45 70.33,85.85 81.92,85.85 84.77,88.71 B1.- | 55.28,61.15 arc45 54.57,60.86 R7-1.1 66.04,72.33 C1.- | R7-2.1 C1.-
N$1
  Bottom 0.508: IC91.3 29.53,10.16 | R93.1 29.46,10.16 29.53,10.16 | R94.2 29.53,10.16
N$2
  Bottom 0.508: R94.1 22.42,6.1 43.81,6.1 45.47,7.37 X7.1
N$3
  Top 0.508: R2.2 98.55,28 98.55,37.27 C2.+
N$4
  Top 2: K1.P 78.23,79.18 | J1.2 78.23,79.12 78.23,79.18 | 78.11,79.06 arc90 78.23,79.18 | B1.AC1 72.2,86.2 72.2,80.77 73.91,79.06 78.11,79.06 | 78.11,79.06 78.23,79.18
N$5
  Bottom 0.508: C2.- D5.A 94.87,28.7 83.76,28.7 81.15,31.31 D6.C
N$6
  Top 0.508: Q3.B 10.6,56.07 15.62,51.05 R19.1
  Bottom 0.508: Q3.B 10.6,60.2 8.83,61.98 4.51,61.98 R20.2
N$7
  Bottom 0.508: R3.1 C3.- D6.A
N$8
  Bottom 0.508: D59.A 5.4,46.67 D60.C
N$9  (via drill 0.35)
  Top 0.508: v15.88,38.1 18.92,35.05 22.42,35.05 D9.C | R20.1 2.73,49.85 4,48.58 4,43.88 2.6,42.48 D59.C
  Bottom 0.508: 2.54,36.45 D59.C 2.6,38.42 3.75,39.56 8.89,39.56 10.35,38.1 v15.88,38.1 | D9.C 22.99,33.91 23.94,32.96 23.94,27.05 23.62,26.73 IC3.6 21.08,26.73 17.27,30.54 12.83,30.54 C8.2
N$10
  Bottom 0.508: D51.C 4.76,23.37 R21.2 8.51,26.35 C8.1 14.86,29.27 IC3.2
N$11
  Top 0.508: X1.1 4.64,17.59 4.06,18.29 4.06,41.59 6.99,44.58 6.99,48.83 5.59,49.78 R22.1
N$12
  Bottom 0.508: R22.2 Q3.C 8.06,56.01 9.08,54.67 12.7,54.67 13.1,54.67 13.84,54.67 14.41,55.24 R28.1
N$13
  Bottom 0.508: D3.C D2.C 88.2,63.69 89.72,62.17 89.72,45.47 87.63,43.37 R55.2 90.36,40.13 C11.+
N$14  (via drill 0.35)
  Top 0.508: v19.05,25.53 19.11,25.46 31.94,25.46 34.73,28.26 X_P2.2
  Bottom 0.508: IC3.3 v19.05,25.53
N$15  (via drill 0.35)
  Top 0.508: v57.34,40.77 55.29,40.77 53.91,39.37 48.01,33.53 v35.94,33.53
  Bottom 0.508: v57.34,40.77 57.34,46.61 R17.2 | v35.94,33.53 32.96,30.54 X_P2.1 32.26,29.21
N$16
  Bottom 0.508: X_P2.3 37.27,28 32.26,21.46 29.84,19.18 24.89,19.18 21.46,22.61 13.14,22.61 12.38,23.37 R18.2
N$17
  Top 0.508: IC1.3 19.94,47.43 19.94,55.24 | 19.94,55.24 18.48,56.71 R6.2 | 19.94,55.24 21.27,56.58 R5.2
N$18
  Bottom 0.508: R43.2 R44.2 9.4,80.01 12.19,80.01 16.26,75.95 16.26,74.1 21.53,68.83 R41.1
N$19
  Bottom 0.508: VR51.3 8.51,51.24 R4.2 8.57,45.97 8.57,44.32 11.68,42.23 IC1.2
N$20
  Top 0.508: J5.1 P1.1
  Top 2: R7-1.2 54.42,30.73 58.99,30.73 | R7-2.2 70.36,30.73 58.99,30.73 | P1.1 58.98,30.72 58.99,30.73
  Bottom 2: R7-1.2 54.51,28.89
N$21
  Bottom 0.508: R9.2 C4.1 25.78,32.96 R8.1
N$22
  Top 0.508: R9.1 28.51,44.39 30.54,42.67 43.12,42.67 Q90.D
  Bottom 0.508: IC2.3 27.62,52.52 25.46,50.36 25.46,48.58 | 25.46,48.58 28.32,45.72 R9.1 | D9.A 25.46,48.2 25.46,48.58
N$23
  Top 0.508: R95.2 27.81,6.1 18.67,6.1 17.4,7.37 17.4,10.98 15.39,12.99 C93.+
  Bottom 0.508: R95.2 IC91.4
N$24
  Bottom 0.508: RV1.S 39.37,52.52 37.91,53.78 36.45,53.78 34.54,52.07 34.48,52.01 34.48,49.4 33.59,48.51 27.5,48.51 26.92,49.09 R10.2
N$25
  Bottom 0.508: IC2.1 32.96,57.59 34.29,56.32 37.85,56.32 38.86,55.05 RV1.E
N$26
  Bottom 0.508: IC2.5 RV1.A
N$27  (via drill 0.35)
  Top 0.508: 51.56,46.67 51.56,39.88 49.3,37.62 Q1.C | 51.56,46.67 51.56,47.13 51.61,47.2 51.56,47.44 51.56,47.82 v49.72,49.66 | 51.56,46.67 51.63,46.61 R15.1
  Bottom 0.508: C9.1 30.16,42.06 30.16,46.42 31.3,47.56 35.69,47.56 | v49.72,49.66 45.72,49.66 43.62,47.56 35.69,47.56 | IC2.6 35.69,50.99 35.69,47.56
N$28
  Top 0.508: R14.2 25.84,41.91 | 25.84,41.91 43.18,41.91 46.99,40.13 Q1.B | R13.1 24.38,48.13 24.38,43.37 25.84,41.91
N$29
  Bottom 0.508: R15.2 59.5,42.93 62.36,45.4 D10.C
  Bottom 1.016: D10.C 62.36,51.43 Q2.3
N$30
  Bottom 0.508: 7.56,73.53 R45.2 7.18,73.53 | R44.1 7.18,73.53 | IC5.2 7.18,74.17 7.18,73.53
N$31
  Bottom 0.508: R26.2 R27.1 IC5.5
N$32
  Top 0.508: IC91.2 36.83,12.7 39.31,10.22 41.78,10.22 IC91.6
  Bottom 0.508: R91.1 R92.2 | IC91.2 32.89,12.7 R92.2 | X2.2 15.81,9.65 17.91,11.68 20.64,11.68 24,16.19 R92.2
N$33
  Bottom 0.508: IC5.3 14.29,76.2 15.18,75.31 RV2.S
N$34  (via drill 0.35)
  Top 0.508: C15.+ 35.56,37.85 35.75,38.04 v41.34,38.04
  Bottom 0.508: v41.34,38.04 41.34,34.92 42.8,33.46 X_P1.2 | C15.+ 34.14,36.58 34.14,36.43 25.4,27.69 R8.2
N$35
  Top 0.508: IC2.2 31.58,53.25 C9.2
  Bottom 0.508: C9.2 34.57,45.72 | 34.57,45.72 R11.2 D58.C 42.67,45.72 R12.2 | C6.1 34.5,45.78 34.57,45.72
N$36
  Bottom 0.508: IC91.5 39.5,7.62 38.29,8.83 C92.1
N$37  (via drill 0.35)
  Top 0.508: R29.1 42.29,74.8 v35.62,74.8
  Bottom 0.508: X5.1 35.62,91.76 38.09,93.97 46.68,93.97 47.88,92.77 47.82,80.26 R29.1 | IC5.6 30.92,76.2 32.32,74.8 v35.62,74.8
N$38
  Top 0.508: X8.2 8.26,63.69 9.21,62.74 R33.2
N$39
  Bottom 0.508: 9.27,83.69 R45.1 11.81,83.69 | R46.1 32.07,66.55 32.07,68.52 | 32.07,68.52 32.07,71.82 28.96,74.93 18.1,74.93 17.34,75.69 17.34,79.06 12.7,83.69 11.81,83.69 | Q41.B 42.99,68.58 32.13,68.58 32.07,68.52 | IC5.1 11.75,83.63 11.81,83.69
N$40
  Top 0.508: RV3.E 34.04,78.61 32.45,78.61 30.42,76.58 R30.1 32.32,70.04 34.23,68.14 34.23,64.71 VR2.R
  Bottom 0.508: VR2.R VR2.C | RV2.E 18.86,67.06 27.88,67.06 30.42,69.6 R30.1
N$41  (via drill 0.35)
  Top 0.508: K1.1 76.33,65.28 59.56,65.28 57.53,67.31 57.53,67.37 v57.47,67.44 | Q41.C 50.29,72.01 v52.32,69.98
  Bottom 0.508: K1.1 84.64,58.33 D41.A | v57.47,67.44 54.8,67.44 52.32,69.91 v52.32,69.98
N$42
  Top 2: Q4.3 56,89.02 53.4,85.85 43.75,85.85 R24.2
N$43
  Top 0.508: 78.87,12.7 82.36,16.19 82.36,24.32 C13.+
  Top 1.016: J6.1 78.87,12.7 X11.1
  Bottom 0.508: C13.+ 86.3,24.32 D1.C
N$44
  Bottom 1.016: R52.2 69.6,24.32 | 69.6,24.32 IC4.1 | R51.2 69.66,24.26 69.6,24.32
N$45
  Bottom 0.508: R26.1 29.4,77.53 31.69,77.53 33.21,76.01 RV3.S
N$46
  Top 0.508: 81.41,73.98 J2.2
  Bottom 1.016: J2.2 83.19,73.98 85.98,71.37 85.98,60.39 86.49,59.88 86.55,59.88 D2.A
  Bottom 2: X4.4 86.36,76.2 86.17,76.01 81.28,76.01 | 81.28,76.01 78.74,76.01 | 78.74,76.01 K1.O | J1.1 78.17,75.44 78.74,76.01 | J2.2 81.53,75.76 81.28,76.01
N$47
  Bottom 2: Q5.3 26.68,90.41 R25.2
N$48
  Bottom 0.508: X13.1 11.49,11.88 R23.1
N$49
  Bottom 0.508: 19.66,52.42 R7.2 | R28.2 19.6,52.4 R7.2 | R7.2 22.68,52.34 23.3,52.96 23.3,54.27 Q7.B
N$50
  Bottom 1.016: Q4.1 45.1,88.98 45.09,86.36 45.15,86.17 | R16.2 arc-45 65.47,48.48 65.64,48.65 67.18,49.72 67.18,56.45 65.72,57.09 Q2.1 54.86,57.28 53.28,58.45 50.99,61.05 50.99,73.66 45.15,78.93 45.15,86.17 | Q5.1 15.55,86.36 45.15,86.17
N$51
  Bottom 0.508: X12.1 84.33,10.03 80.71,13.78 C14.+ 83.63,20.19 88.2,20.19 D4.C
N$52  (via drill 0.35)
  Top 0.508: v91.44,52.26 91.38,52.26 89.92,50.8 89.92,42.35 87.88,40.32 87.88,35.37 88.71,34.54 88.71,28.13 87.06,26.48 87.06,15.94 D1.A
  Bottom 0.508: v91.44,52.26 91.44,58.99 92.16,59.71 X10.4
N$53
  Bottom 0.508: X2.1 13.27,8.95 17.4,13.08 18.1,13.78 18.44,14.12 | C91.+ 15.3,17.65 18.44,14.12 | 18.44,14.12 R93.2
N$54  (via drill 0.35)
  Top 0.508: v7.11,41.78 7.11,28.45 11.43,24.13 R23.2
  Bottom 0.508: Q7.C 25.46,55.18 25.46,52.77 23.18,50.48 15.49,50.48 12.51,53.66 8.19,53.66 7.11,52.58 v7.11,41.78
N$55
  Top 0.508: D4.A 93.98,15.75 93.98,39.81 97.22,43.12 97.22,47.94 95.25,49.72 X10.2
N$56  (via drill 0.35)
  Top 0.508: R33.1 33.27,62.74 35.3,60.7 | 35.3,60.7 35.33,60.68 | 35.3,60.7 40.58,60.7 v42.86,58.42
  Bottom 0.508: v42.86,58.42 45.78,58.42 47.62,56.64 Q6.C
N$57
  Top 0.508: C13.- 80.77,30.48 82.93,32.64 82.93,40.51 85.34,42.93 85.34,49.34 90.87,54.86 93.8,54.86 X10.3
  Bottom 0.508: C13.- 78.74,24.26 78.74,12.7 79.18,12.26
  Bottom 1.016: J7.1 79.18,12.26 81.41,10.03 X11.2
N$59  (via drill 0.35)
  Top 0.508: X10.1 92.9,43.6 92.9,28.13 90.61,25.84 v90.61,20.57
  Bottom 0.508: X12.2 86.87,10.03 84.26,12.83 C14.- 87.12,17.27 v90.61,20.57
N$60
  Bottom 0.508: D41.C 78.61,60.52 81.36,63.26 D42.C
OUT+  (1 unrouted)
  Top 0.508: D11.C 41.53,17.46 40.26,18.73 40.26,21.08 U_METER.1
  Bottom 0.508: P2.1 60.07,10.16 J3.2 59.31,10.67 OUT+.1 | R41.2 27.5,83.88
  Bottom 1.016: 51.5,34.54 60.52,34.54 61.4,35.43 C57.2 | R16.1 D10.A 61.98,36.9 C57.2 | C7.+ C57.2
  Bottom 2: P2.1 57.21,17.4 51.74,17.4 51.68,17.46 D11.C 51.44,17.43 51.5,21.11 51.5,34.54 52.32,35.43 52.32,56.58 52.23,56.99 52.02,57.21 48.91,60.32 48.91,72.56 48.77,72.71 42.24,78.71 42.24,82.03 R24.1 R25.1
OUT-  (via drill 0.35)
  Top 0.508: U_METER.2 43.56,20.32 49.85,20.32 51.56,18.61 v51.56,15.68
  Bottom 0.508: 68.39,10.53 68.01,10.15 68.01,8.19 67.5,7.68 J4.1 OUT-.1 v51.56,15.68 | J5.2 63.5,25.67 | 63.5,25.4 63.5,25.67 | 63.5,25.67 62.93,26.24
  Bottom 1.016: C57.1 64.77,33.34 C7.- 62.93,31.5 62.93,26.24 63.31,25.86
  Bottom 2: D11.A 62.94,17.83 | D11.A 68.45,12.32 68.45,11.94 68.39,10.53 P2.2 | D11.A 63.31,25.86 P1.2
SENSE+
  Bottom 0.508: C6.2 34.8,40.89 39.88,40.89 42.74,38.1 R12.1 44.07,34.29 44.07,27.05 44.96,26.16 44.96,15.24 52.07,8.13 | 52.07,8.13 X6.1 | J3.1 53.59,10.67 52.07,9.14 52.07,8.13
SENSE-
  Top 0.508: R4.1 10.16,38.23 10.16,45.47 12.26,47.56 17.08,47.56 R6.1
  Bottom 0.508: R4.1 R21.1 5.21,33.21 D51.A | J4.2 54.55,7.68 X6.2 54.67,7.56 54.67,6.03 53.98,5.33 51.24,5.33 49.84,6.8 49.84,8.52 44.01,14.29 44.01,16.07 41.47,18.61 41.47,26.23 40.26,27.43 X_P1.1 D58.A 37.21,35.56 | R11.1 37.21,35.56 | R11.1 37.08,35.62 | 31.62,38.1 34.92,38.1 37.08,35.62 | R4.1 D60.A | 37.08,35.62 36.89,35.69 37.21,35.56 | C15.- 31.62,38.1 | 11.87,36.58 IC1.4 | R4.1 8.76,36.83 IC1.4 | IC1.4 16.76,36.83 18.03,38.1 31.62,38.1 | C4.2 28.57,29.27 34.04,34.73 36.26,34.73 R11.1
SHUTDOWN  (via drill 0.35)
  Top 0.508: v29.91,79.18 29.91,77.72 29.25,77.06 29.25,62.2 31.95,59.5 v36.07,59.5 | IC91.7 49.66,12.7 53.08,15.44 53.15,15.49 53.15,19.24 49.53,22.86 R90.2 49.47,22.99 OFF.1
  Bottom 0.508: R90.2 49.4,31.12 48.07,32.45 48.07,33.59 50.61,36.32 50.61,46.67 | IC5.7 19.56,78.74 20.73,77.57 23.98,77.57 R27.2 26.73,80.39 28.7,80.39 v29.91,79.18 | v36.07,59.5 46.93,59.5 50.35,56.13 50.61,55.88 50.61,53.72 | 50.61,53.72 50.61,46.67 | Q90.G 50.61,46.67 | Q6.B 50.61,53.72
V+  (via drill 0.4)
  Top 0.508: 56.01,66.86 55.88,66.99 | v74.87,66.86 60.13,66.86 56.96,70.04 56.96,72.58 C1.+ | R13.2 26.67,61.47 26.67,80.14 27.75,81.22 29.46,81.22 30.61,82.36 30.61,86.11 | 30.61,86.68 30.61,86.11 | 30.61,86.11 30.48,85.98 | V+.1 22.48,85.98
  Top 1.016: C1.+ 55.88,66.99 58.9,63.98 61.94,63.98 68.96,56.96 | 73.28,19.05 IC4.3 74.17,19.18 75.95,19.18 76.71,19.94 76.71,27.59 79.29,29.15 79.29,33.27 76.24,33.82 70.42,39.7 70.42,55.5 68.96,56.96 | Q2.2 66.93,54.93 68.96,56.96
  Top 2: Q5.2 20.13,85.98 22.48,85.98 30.48,85.98 31.94,85.98 arc14 33.08,85.92 37.91,81.09 44.64,81.09 46.55,82.99 50.48,82.99 C1.+ 70.1,88.96 B1.+
  Bottom 0.508: R1-2.2 59.05,76.68 55.88,73.51 C1.+ | R1.2 75.88,66.86 v74.87,66.86
  Bottom 1.016: X3.1 73.28,19.05 73.47,19.24 IC4.3 76.88,19.24 C12.1
  Bottom 1.27: C5.1 C1.+
  Bottom 2: Q4.2 50.55,78.23 C1.+
VREF
  Top 0.508: R18.1 11.68,33.53 14.61,36.45 14.61,38.86 16.45,40.7 18.41,40.7 IC1.6
  Bottom 0.508: VR51.1 VR51.2 10.6,48.51 11.68,47.56 19.88,47.56 R5.1 21.27,39.37 | IC1.6 21.27,39.37 | 21.27,39.37 32.32,39.37 32.96,40.07 32.96,41.15 33.72,41.91 40.32,41.91 44.01,38.29 45.09,37.21 45.09,29.53 45.34,29.34 X_P1.3
VSS  (via drill 0.35)
  Top 0.508: 28.51,48.26 29.53,49.28 IC2.4 26.86,52.7 R10.1 | 28.51,48.26 26.04,45.78 25.91,45.59 R14.1 | v48.01,35.75 48.96,35.75 55.05,41.85 65.72,41.85 69.79,37.78 v70.1,37.4 | v32.96,44.07 31.11,44.07 30.1,45.09 30.1,46.74 28.51,48.26 | IC3.4 18.73,28 26.73,28 30.35,31.62 v46.1,31.62
  Bottom 0.508: 31.05,50.36 31.1,50.43 | 31.1,50.43 C52.2 | 31.1,50.43 30.64,49.97 IC2.4 | v48.01,35.75 46.61,35.75 | 46.61,35.75 46.1,35.75 46.1,37.72 40.77,42.99 34.04,42.99 v32.96,44.07 | v46.1,31.62 46.1,35.69 46.61,35.75 | v70.1,37.4 70.1,35.88 71.56,34.42 73.79,34.42 R3.2 | VSS.1 75.88,36.64 R3.2 | R3.2 D7.A

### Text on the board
tNames: Temp. / Fühler | 12V~ | Temp / Schwelle | Relais / Schwelle | Over Temp | 12V~ | Aux ~ | Offset | Aux ~ | Poti I | Poti U | CC | CV | LNG BG v2.11 | Standby | 15.01.2018 | Standby | Out | 30V Aux | 9V Aux | 9V Aux | Sense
